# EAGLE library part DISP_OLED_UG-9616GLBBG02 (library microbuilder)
96x16 0.84" I2C Mono OLED Display
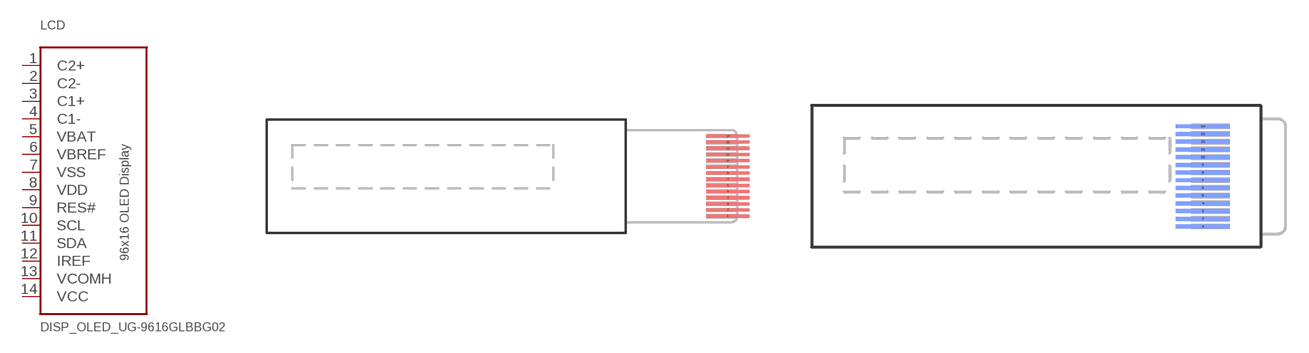
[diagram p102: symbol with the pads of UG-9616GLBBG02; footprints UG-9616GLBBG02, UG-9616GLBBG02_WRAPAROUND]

Designator prefix LCD

## DISP_OLED_UG-9616GLBBG020.5MMFLAT  [UG-9616GLBBG02]
1  C2+
2  C2-
3  C1+
4  C1-
5  VBAT
6  VBREF
7  VSS
8  VDD
9  RES#
10  SCL
11  SDA
12  IREF
13  VCOMH
14  VCC

## DISP_OLED_UG-9616GLBBG020.5MMWRAPUNDER  [UG-9616GLBBG02_WRAPAROUND]
Pads as for UG-9616GLBBG02

## DISP_OLED_UG-9616GLBBG02  [UG-9616GLBBG02_0.65MM_WRAPAROUND]
Pads as for UG-9616GLBBG02

## Footprint UG-9616GLBBG02 (pad centres in mm)
96x16 OLED Display - 0.84"/29.1x9.2mm
smd 3.5 x 0.254: 1 8.25,-3.25; 2 8.25,-2.75; 3 8.25,-2.25; 4 8.25,-1.75; 5 8.25,-1.25; 6 8.25,-0.75; 7 8.25,-0.25; 8 8.25,0.25; 9 8.25,0.75; 10 8.25,1.25; 11 8.25,1.75; 12 8.25,2.25; 13 8.25,2.75; 14 8.25,3.25

## Footprint UG-9616GLBBG02_WRAPAROUND (pad centres in mm)
smd 3.5 x 0.254 bottom: 1 -3.75,-3.25; 2 -3.75,-2.75; 3 -3.75,-2.25; 4 -3.75,-1.75; 5 -3.75,-1.25; 6 -3.75,-0.75; 7 -3.75,-0.25; 8 -3.75,0.25; 9 -3.75,0.75; 10 -3.75,1.25; 11 -3.75,1.75; 12 -3.75,2.25; 13 -3.75,2.75; 14 -3.75,3.25

## Footprint UG-9616GLBBG02_0.65MM_WRAPAROUND (pad centres in mm)
smd 3.5 x 0.3 bottom: 1 -5.75,-4.225; 2 -5.75,-3.575; 3 -5.75,-2.925; 4 -5.75,-2.275; 5 -5.75,-1.625; 6 -5.75,-0.975; 7 -5.75,-0.325; 8 -5.75,0.325; 9 -5.75,0.975; 10 -5.75,1.625; 11 -5.75,2.275; 12 -5.75,3.575; 13 -5.75,2.925; 14 -5.75,4.225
